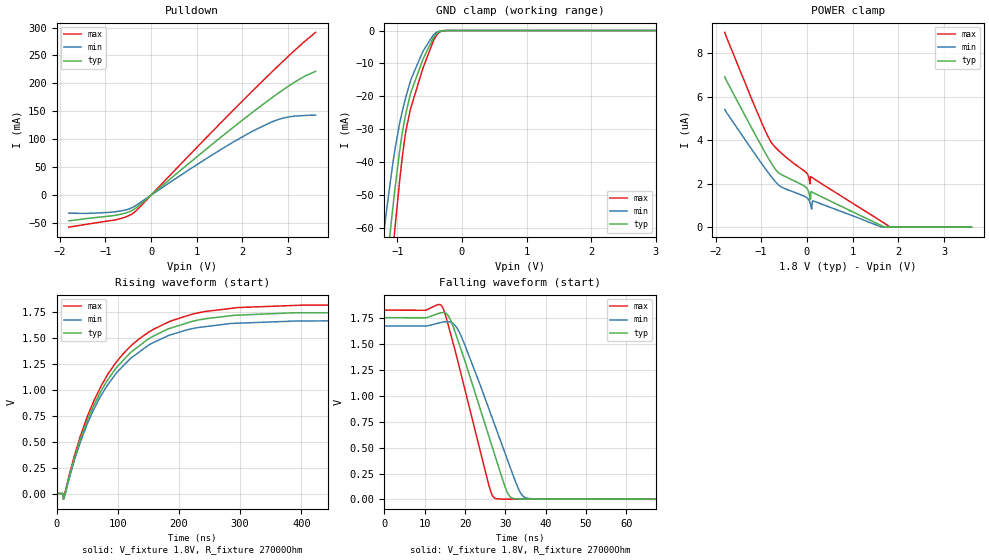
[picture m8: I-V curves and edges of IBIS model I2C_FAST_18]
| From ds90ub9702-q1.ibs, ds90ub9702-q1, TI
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|   I2C_Fast_18 Model
[Model]   I2C_FAST_18
Model_type   I/O_open_drain
Polarity   Non-Inverting
Enable   Active-High
Vinl = 0.54
Vinh = 1.26
Vmeas = 0.9
Vref = 1.8
Cref = 0pF
Rref = 27000
|   typ   min   max
C_comp   1.3293528pF  1.3920023pF  1.3293528pF
[Voltage Range]   1.8   1.71   1.89
[Temperature Range]   27   105   -40
[Pullup Reference]   1.8   1.71   1.89
[Pulldown Reference]   0   0   0
[Power Clamp Reference]   1.8   1.71   1.89
[GND Clamp Reference]   0   0   0
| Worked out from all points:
|   slope of the pulldown table from 0 to 0.27 V, typ, clamps not added: 14.5 ohm
|   GND clamp passes 1 mA (typ) near -0.39 V on its own axis
|   falling waveform, V_fixture 1.8V, R_fixture 27000Ohm: 20-80 % time 8.63ns typ, 9.53ns min, 7.06ns max; typ from 1.75 V to 0.001 V
|   rising waveform, V_fixture 1.8V, R_fixture 27000Ohm: 20-80 % time 100ns typ, 98.7ns min, 99ns max; typ from 0.001 V to 1.75 V
[Pulldown]
|   Voltage   I(typ)   I(min)   I(max)
-1.8V     -46.05mA   -32.39mA   -57.33mA
-1.39V    -41.67mA   -32.67mA   -51.89mA
-801mV    -36.39mA   -29.97mA   -44.68mA
-531mV    -31.37mA   -25.98mA   -38.26mA
-369mV    -25.03mA   -20.3mA    -30.81mA
1.219V    83.16mA    65.87mA    103.7mA
1.796V    121.2mA    94.83mA    151.9mA
2.266V    151.2mA    116.4mA    190.4mA
2.628V    173.3mA    130.5mA    219.4mA
2.909V    189.7mA    138.3mA    241.3mA
3.357V    212.7mA    142.6mA    274.8mA
3.6V      221.6mA    143.2mA    291.5mA
[GND Clamp]
|   Voltage   I(typ)   I(min)   I(max)
-1.8V     -199.4mA   -169.6mA   -233.1mA
-1.217V   -81.45mA   -62.71mA   -99.08mA
-1.195V   -77.25mA   -59.17mA   -94.26mA
-1.163V   -71.03mA   -53.98mA   -87.07mA
-1.071V   -54.02mA   -40.47mA   -67.16mA
-1.039V   -48.35mA   -36.29mA   -60.36mA
-919.8mV  -30.64mA   -24.24mA   -37.84mA
-865.8mV  -24.89mA   -19.99mA   -30.25mA
-801mV    -19.58mA   -15.58mA   -24.22mA
-595.8mV  -8.39mA    -6.051mA   -11mA
-390.6mV  -916.2uA   -527.9uA   -1.415mA
3.6V      0A         0A         0A
[POWER Clamp]
|   Voltage   I(typ)   I(min)   I(max)
-1.8V     6.905uA    5.414uA    8.951uA
-790.2mV  2.974uA    2.348uA    3.928uA
-606.6mV  2.475uA    1.914uA    3.491uA
-12.6mV   1.815uA    1.368uA    2.501uA
36mV      1.629uA    1.267uA    2.314uA
68.4mV    1.266uA    1.118uA    1.987uA
79.2mV    1.285uA    1.038uA    2.319uA
84.6mV    1.557uA    989.8nA    2.319uA
100.8mV   1.623uA    827nA      2.295uA
133.2mV   1.587uA    1.209uA    2.25uA
1.818V    0A         0A         1.266nA
3.6V      0A         0A         0A
[Ramp]
R_load = 27000
|   typ   min   max
dV/dt_r   1.05129/9.92072e-08   1.00331/9.7764e-08   1.09497/9.88903e-08
dV/dt_f   1.05146/8.62781e-09   1.00337/9.52236e-09   1.09514/7.0585e-09
[Falling Waveform]
V_fixture = 1.8V
V_fixture_min = 1.71V
V_fixture_max = 1.89V
R_fixture = 27000Ohm
C_fixture = 0F
|   Time   V(typ)   V(min)   V(max)
0s        1.753V     1.673V     1.826V
14.32ns   1.802V     1.709V     1.861V
15.93ns   1.766V     1.715V     1.668V
18.45ns   1.51V      1.623V     1.297V
26.46ns   542.2mV    816.4mV    67.93mV
29.08ns   222.3mV    537.6mV    2.583mV
31.15ns   27.34mV    316.1mV    2.26mV
33.94ns   3.19mV     52.75mV    2.164mV
38.91ns   2.946mV    3.425mV    1.993mV
1.25us    961.3uV    1.134mV    814.6uV
[Rising Waveform]
V_fixture = 1.8V
V_fixture_min = 1.71V
V_fixture_max = 1.89V
R_fixture = 27000Ohm
C_fixture = 0F
|   Time   V(typ)   V(min)   V(max)
0s        961.3uV    1.134mV    814.6uV
10.17ns   953.2uV    1.123mV    817.4uV
11.24ns   -41.76mV   -7.329mV   -55.23mV
12.23ns   -40.28mV   -47.44mV   -31.69mV
48.93ns   685.5mV    653.7mV    722.7mV
95.35ns   1.196V     1.146V     1.252V
151.2ns   1.497V     1.436V     1.562V
221.2ns   1.663V     1.592V     1.732V
403.8ns   1.746V     1.667V     1.82V
1.25us    1.753V     1.673V     1.826V
